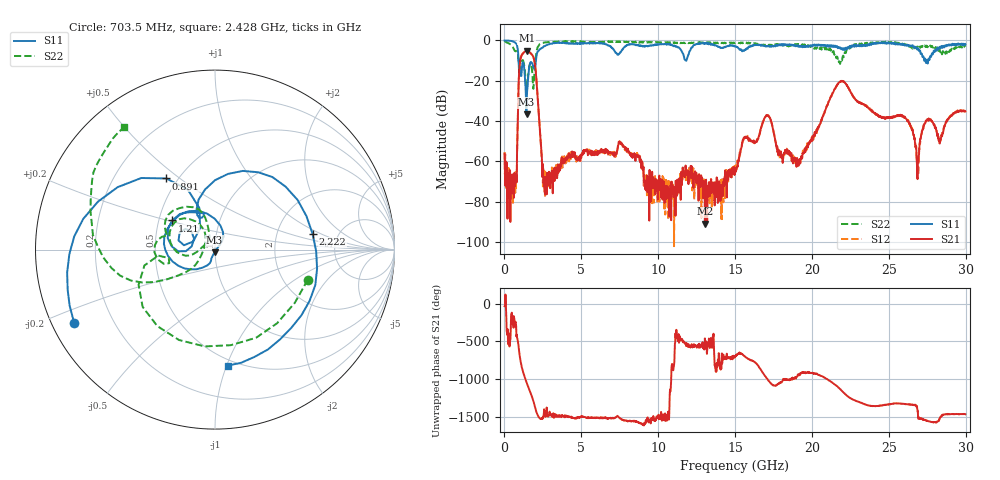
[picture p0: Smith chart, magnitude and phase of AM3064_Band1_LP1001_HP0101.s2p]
# Hz S DB R 50.0
!freq dBS11 angS11 dBS21 angS21 dBS12 angS12 dBS22 angS22
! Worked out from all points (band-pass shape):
!   1600 points, 10 MHz to 29.98 GHz, reference 50 ohm
!   highest |S21| = -5.13 dB at 1.453 GHz (marker M1); lowest = -90.9 dB at 13.04 GHz (marker M2)
!   |S21| within 3 dB of the highest: 1.081 GHz to 1.87 GHz (788.8 MHz wide, 53.5 % of centre)
!   lowest |S11| = -36.7 dB at 1.435 GHz (marker M3), VSWR 1.03, Z = 49.7 - j1.43 ohm
!   |S11| at or under -10 dB: 916.7 MHz to 2.044 GHz (1.127 GHz wide, 76.2 % of centre); 27.39334 GHz to 27.45989 GHz (66.55 MHz wide, 0.243 % of centre); 27.49012 GHz to 27.56345 GHz (73.32 MHz wide, 0.266 % of centre)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
!   |S22| runs from -24.6 to -0.3 dB; largest |S21 - S12| = 0.0065
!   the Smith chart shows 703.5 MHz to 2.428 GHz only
!   S11 on the Smith chart (normalised r, x): 703.5 MHz: 0.06, -0.24; 891 MHz: 0.43, +0.45; 1.21 GHz: 0.59, +0.21; 2.222 GHz: 3.23, +0.81; 2.428 GHz: 0.45, -1.01
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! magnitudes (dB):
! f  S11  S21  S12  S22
! 10 MHz  0.0  -56.2  -55.4  -0.3
! 703.5 MHz  -1.1  -71.2  -75.6  -5.3
! 891 MHz  -6.4  -30.0  -30.0  -7.9
! 1.21 GHz  -10.8  -6.5  -6.4  -9.9
! 1.435 GHz  -36.7  -5.2  -5.1  -24.6
! 1.453 GHz  -29.0  -5.1  -5.1  -24.4
! 2.222 GHz  -5.2  -35.1  -34.9  -2.6
! 2.428 GHz  -3.7  -57.4  -59.8  -1.4
! 2.69 GHz  -2.5  -68.3  -69.7  -0.9
! 5.015 GHz  -1.4  -57.4  -56.5  -0.6
! 7.582 GHz  -5.6  -50.7  -50.8  -0.5
! 10 GHz  -2.0  -73.5  -69.4  -0.9
! 13.04 GHz  -1.6  -90.9  -69.9  -1.2
! 15 GHz  -2.9  -64.8  -66.0  -1.4
! 17.05 GHz  -2.8  -37.1  -37.2  -2.7
! 18.06 GHz  -2.1  -57.7  -57.8  -1.9
! 19.99 GHz  -2.9  -48.5  -49.4  -3.0
! 21.88 GHz  -4.0  -20.4  -20.4  -9.7
! 25 GHz  -1.1  -38.2  -38.3  -1.1
! 26.87 GHz  -4.3  -68.8  -65.4  -3.2
! 27.49 GHz  -9.9  -39.7  -39.3  -3.1
! 29.98 GHz  -1.8  -35.3  -35.3  -3.1
